(* Logix 5000 AddOnInstructionDefinition export; software revision 16.00 *)

ADD_ON_INSTRUCTION SCP   (* revision 1.2, vendor Rockwell Automation *)
// Scale w/Parameters
// Help:
// Use this instruction to scale data from your analog module and bring it into the limits prescribed by the process variable or another analog module.
// Equations used in calculating a linear relationship:
// Scaled value = (input value - input min.) x rate + scaled minimum
// Rate = (scaled max. - scaled min.) / (input max. - input min.)
VAR_INPUT
   Input : REAL; {required}
   Input_Min : REAL; {required}
   Input_Max : REAL; {required}
   Scaled_Min : REAL; {required}
   Scaled_Max : REAL; {required}
END_VAR
VAR_OUTPUT
   Output : REAL; {required}
END_VAR
VAR
   Rate : REAL;
END_VAR

ROUTINE Logic   (* ladder *)
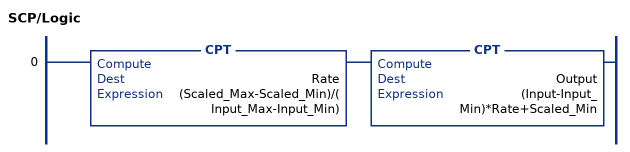
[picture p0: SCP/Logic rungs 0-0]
   0: CPT(Rate,(Scaled_Max-Scaled_Min)/(Input_Max-Input_Min))CPT(Output,(Input-Input_Min)*Rate+Scaled_Min);
END_ROUTINE
END_ADD_ON_INSTRUCTION
